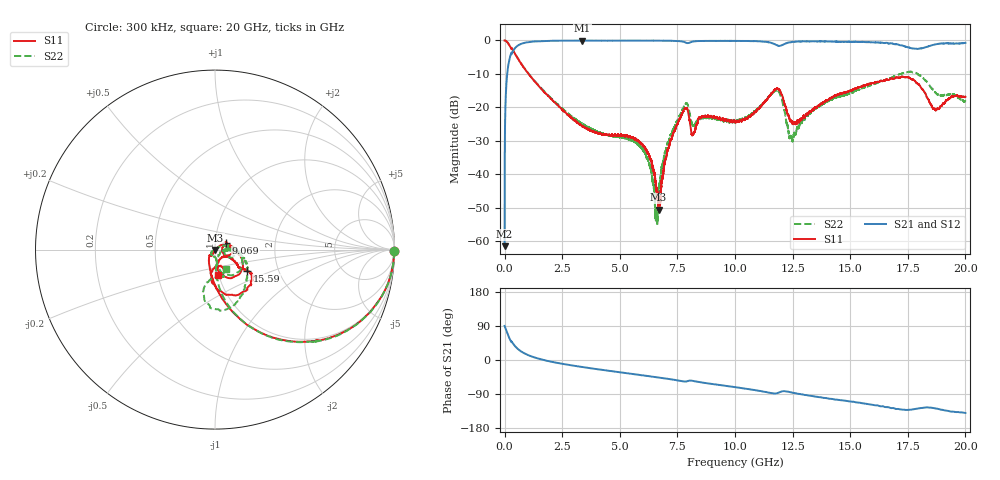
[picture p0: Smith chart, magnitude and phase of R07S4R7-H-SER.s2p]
!{R07S4R7}
!Johanson Technology Inc.
!www.johansontechnology.com
!Test Board Conditions:
!Substrate Type  RO4350B
!Substrate Thickness  10 mil
!Substrate Dk  3.66
!TL Type: GCPW
!TL Trace Width  21 mil
!TL Gap  20 mil
!Electrode orientation  Horizontal
!DUT TOPOLOGY	SERIES
!Mounting Pad LxW  16x21 mil
! Created Sat Feb  6 11:34:19 2021
# hz S ma R 50
! 2 Port Network Data from SP1.SP block
! freq  magS11  angS11  magS21  angS21  magS12  angS12  magS22  angS22
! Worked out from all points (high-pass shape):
!   20001 points, 300 kHz to 20 GHz, reference 50 ohm
!   highest |S21| = -0.04 dB at 3.374 GHz (marker M1); lowest = -61.4 dB at 300 kHz (marker M2)
!   |S21| within 3 dB of the highest: 374.5 MHz to end of sweep
!   lowest |S11| = -50.5 dB at 6.683 GHz (marker M3), VSWR 1.01, Z = 50.2 - j0.2 ohm
!   |S11| at or under -10 dB: 1.04 GHz to end of sweep
!   |S22| runs from -55.4 to 0.0 dB; largest |S21 - S12| = 0.014
!   S11 on the Smith chart (normalised r, x): 300 kHz: open; 9.069 GHz: 1.13, +0.09; 15.59 GHz: 1.39, -0.34; 20 GHz: 0.99, -0.29
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300000  0.999 -0.5  0.0008501 90.0  0.0008038 90.1  1 -0.6
1.153e8  0.9453 -19.5  0.3213 70.8  0.3218 70.7  0.9456 -19.5
3.413e8  0.7348 -44.2  0.6704 45.4  0.6711 45.4  0.7356 -44.3
1.1173e9  0.2924 -79.9  0.9527 10.6  0.9528 10.5  0.2959 -78.2
3.3343e9  0.05394 -127.5  0.9941 -18.2  0.9942 -18.2  0.05848 -82.0
3.3743e9  0.05198 -129.3  0.9951 -18.6  0.9938 -18.5  0.05676 -81.7
5.8853e9  0.02987 -117.3  0.9939 -39.7  0.9939 -39.7  0.02596 -140.7
6.6673e9  0.003929 -63.3  0.9926 -46.1  0.9924 -46.2  0.003849 47.4
6.6833e9  0.002985 -41.8  0.992 -46.2  0.9931 -46.3  0.005237 54.8
7.0063e9  0.01741 37.7  0.9897 -49.1  0.9889 -49.1  0.02309 31.5
7.8043e9  0.09456 10.9  0.9462 -56.8  0.9456 -56.9  0.1071 5.2
8.1773e9  0.03977 0.7  0.9631 -55.2  0.9629 -55.3  0.05359 -12.2
9.0693e9  0.07259 31.8  0.9855 -63.9  0.9845 -64.0  0.07067 11.8
1.00003e10  0.06173 28.6  0.9857 -71.7  0.9853 -71.8  0.06051 -1.2
1.17983e10  0.1908 -42.1  0.855 -88.0  0.8521 -88.1  0.1822 -40.4
1.24373e10  0.06346 -66.8  0.9434 -85.4  0.9422 -85.6  0.03724 -42.6
1.33343e10  0.09088 -28.3  0.9702 -95.0  0.9705 -95.1  0.08836 2.3
1.55883e10  0.2131 -33.2  0.9467 -114.6  0.9465 -114.6  0.1987 -26.1
1.66673e10  0.2567 -37.3  0.8995 -124.8  0.9037 -125.3  0.2681 -51.6
1.77383e10  0.2599 -76.4  0.7595 -130.1  0.7583 -129.9  0.3325 -88.6
1.86723e10  0.09396 -82.2  0.8702 -127.4  0.8696 -127.3  0.1698 -99.3
2e10  0.1439 -83.8  0.9197 -139.7  0.9158 -139.7  0.1255 -59.6
